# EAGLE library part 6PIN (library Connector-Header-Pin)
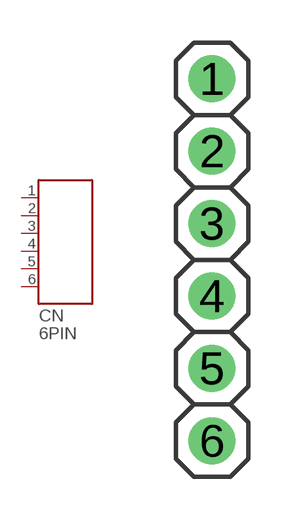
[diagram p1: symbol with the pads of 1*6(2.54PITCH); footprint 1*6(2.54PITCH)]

Designator prefix CN

## 6PIN2.54  [1*6(2.54PITCH)]
1  1
2  2
3  3
4  4
5  5
6  6

## Footprint 1*6(2.54PITCH) (pad centres in mm)
drill 1.1: 1 0,6.35; 2 0,3.81; 3 0,1.27; 4 0,-1.27; 5 0,-3.81; 6 0,-6.35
